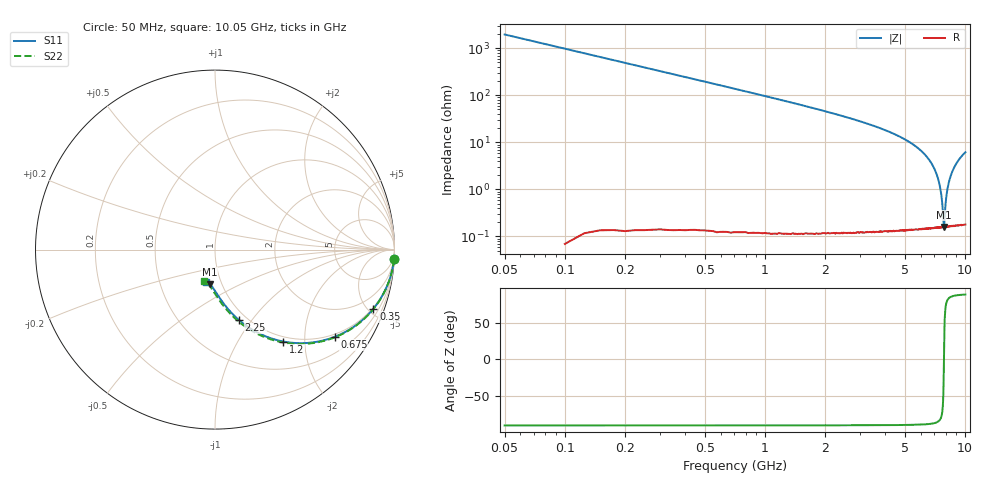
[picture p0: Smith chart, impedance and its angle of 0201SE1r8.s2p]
! AVX Thin Film Operation		Date: August 2001
! Description: Accu-P® Series, Thin Film, SMD, RF Capacitor
! Part Number: 02013J1R8ABW
! 50 MHz  -  10.05 GHz
! Serial Measurements
# mhz S db R 50
!	S11		S21		S12		S22
!	dB	Phase	dB	Phase	dB	Phase	dB	Phase
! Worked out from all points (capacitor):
!   401 points, 50 MHz to 10.05 GHz, reference 50 ohm
!   read as one part in series: C = 1.62 pF near 100 MHz
!   lowest |Z| = 158 mohm at 7.85 GHz (marker M1)
!   series resonance near 7.851 GHz, so ESL is about 250 pH
!   S11 on the Smith chart (normalised r, x): 50 MHz: 1, -38; 350 MHz: 0.92, -5.38; 675 MHz: 0.92, -2.80; 1.2 GHz: 0.92, -1.59; 2.25 GHz: 0.92, -0.87; 10.05 GHz: 0.85, -0.32
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50  -0.01 -3.0  -25.87 86.9  -25.87 86.9  -0.01 -3.1
75  -0.03 -4.6  -22.37 85.4  -22.37 85.4  -0.03 -4.6
125  -0.07 -7.6  -17.98 82.4  -17.98 82.4  -0.07 -7.6
175  -0.14 -10.6  -15.12 79.4  -15.12 79.4  -0.14 -10.6
250  -0.27 -14.9  -12.16 75.0  -12.16 75.0  -0.27 -15.1
350  -0.52 -20.5  -9.49 69.4  -9.49 69.4  -0.52 -20.7
425  -0.74 -24.5  -8.04 65.4  -8.04 65.4  -0.74 -24.7
500  -1.00 -28.2  -6.88 61.6  -6.88 61.6  -1.00 -28.5
675  -1.67 -36.1  -4.97 53.6  -4.97 53.6  -1.67 -36.5
900  -2.62 -44.6  -3.45 45.1  -3.45 45.1  -2.62 -45.1
1200  -3.90 -53.4  -2.28 36.2  -2.28 36.2  -3.90 -54.0
1450  -4.91 -59.0  -1.70 30.5  -1.70 30.5  -4.91 -59.8
1725  -5.93 -64.0  -1.29 25.4  -1.29 25.4  -5.94 -65.0
2250  -7.62 -71.1  -0.84 18.1  -0.84 18.1  -7.62 -72.3
2750  -8.94 -76.0  -0.60 13.1  -0.60 13.1  -8.94 -77.5
3400  -10.31 -80.8  -0.44 8.1  -0.44 8.1  -10.31 -82.7
4175  -11.56 -85.2  -0.33 3.4  -0.33 3.4  -11.56 -87.5
5050  -12.59 -89.2  -0.26 -0.8  -0.26 -0.8  -12.60 -91.9
6725  -13.80 -95.2  -0.20 -7.4  -0.20 -7.4  -13.82 -98.7
7850  -14.25 -98.7  -0.18 -11.2  -0.18 -11.2  -14.27 -102.7
8400  -14.39 -100.3  -0.17 -12.9  -0.17 -12.9  -14.41 -104.6
10050  -14.60 -104.8  -0.17 -17.9  -0.17 -17.9  -14.62 -109.8
